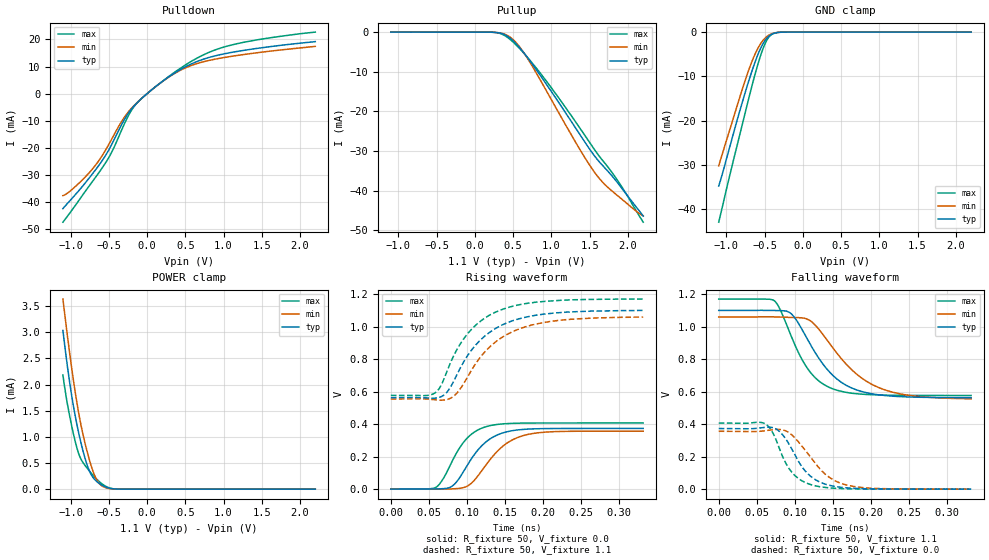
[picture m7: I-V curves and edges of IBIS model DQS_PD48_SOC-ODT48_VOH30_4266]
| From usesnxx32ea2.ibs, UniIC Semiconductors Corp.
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| DQS_PD48_SOC-ODT48_VOH30_4266
| (48 Ohm Pulldown, 48 Ohm System ODT Setting, VOH=VDDQ/3.0, 3200-4266Mbps)
[Model]   DQS_PD48_SOC-ODT48_VOH30_4266
Model_type   I/O
Vinl = 123.333mV
Vinh = 243.333mV
Vmeas = 183.333mV
Vref = 0.0mV
Cref = 0.0pF
Rref = 48.000Ohm
|   typ   min   max
|C_comp   0.849pF   0.799pF   0.899pF
C_comp_pullup   0.4245pF   0.3995pF   0.4495pF
C_comp_pulldown   0.4245pF   0.3995pF   0.4495pF
| Note: C_comp changes when the ODT circuit is enabled.
[Model Spec]
| Input threshold voltage corners
Vinl   0.1233V   0.1167V   0.1350V
Vinh   0.2433V   0.2367V   0.2550V
| Measurement voltage corners
Vmeas   0.1833V   0.1767V   0.1950V
| Timing spec test load voltage corners
Vref   0.0000V   0.0000V   0.0000V
| Dynamic Overshoot Parameters from LPDDR4 Specification
D_overshoot_ampl_h   0.30   NA   NA
D_overshoot_ampl_l   0.30   NA   NA
D_overshoot_area_h   0.1n   NA   NA
D_overshoot_area_l   0.1n   NA   NA
[Voltage Range]   1.1000V   1.0600V   1.1700V
[Pullup Reference]   1.1000V   1.0600V   1.1700V
| Junction Temperature (Ambient temp is 35C typ 95C min -40C max)
[Temperature Range]   50.0   110.0   -40.0
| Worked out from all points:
|   slope of the pulldown table from 0 to 0.165 V, typ, clamps not added: 43.9 ohm
|   slope of the pullup table from 0 to 0.165 V, typ, clamps not added: 15.7 kohm
|   GND clamp passes 1 mA (typ) near -0.45 V on its own axis
|   POWER clamp passes 1 mA (typ) near -0.88 V on its own axis
|   rising waveform, R_fixture 50, V_fixture 0.0: 20-80 % time 36.2ps typ, 40.6ps min, 31.9ps max; typ from 0.001 V to 0.373 V
|   falling waveform, R_fixture 50, V_fixture 1.1: 20-80 % time 49.2ps typ, 61ps min, 39.1ps max; typ from 1.1 V to 0.563 V
|   rising waveform, R_fixture 50, V_fixture 1.1: 20-80 % time 55.7ps typ, 58.6ps min, 51.8ps max; typ from 0.563 V to 1.1 V
|   falling waveform, R_fixture 50, V_fixture 0.0: 20-80 % time 32.4ps typ, 39.9ps min, 27.4ps max; typ from 0.373 V to 0.001 V
[Pulldown]
|   Voltage   I(typ)   I(min)   I(max)
-1.1V     -42.4mA    -37.62mA   -47.4mA
-911.9mV  -36.43mA   -33.59mA   -40.22mA
-680.9mV  -28.37mA   -26.64mA   -31.14mA
-482.9mV  -19.86mA   -17.85mA   -22.71mA
-314.6mV  -10.51mA   -9.476mA   -12.3mA
-176mV    -4.726mA   -4.587mA   -5.011mA
-47.3mV   -1.184mA   -1.177mA   -1.166mA
266.2mV   5.832mA    5.742mA    5.954mA
589.6mV   11.09mA    10.5mA     12.08mA
965.8mV   14.43mA    13.11mA    16.84mA
1.444V    16.71mA    15.1mA     19.86mA
2.2V      19.18mA    17.44mA    22.7mA
[GND Clamp]
|   Voltage   I(typ)   I(min)   I(max)
-1.1V     -34.74mA   -30.2mA    -42.91mA
-948.2mV  -25.43mA   -21.63mA   -31.79mA
-796.4mV  -16.11mA   -13.14mA   -21.19mA
-723.8mV  -11.93mA   -9.348mA   -16.1mA
-661.1mV  -8.566mA   -6.435mA   -11.85mA
-588.5mV  -5.112mA   -3.681mA   -7.299mA
-522.5mV  -2.666mA   -1.902mA   -3.81mA
-469.7mV  -1.356mA   -992.7uA   -1.786mA
-413.6mV  -564.8uA   -417.5uA   -621.5uA
-350.9mV  -166uA     -126.7uA   -147.9uA
-235.4mV  -8.3uA     -7.759uA   -4.464uA
2.2V      0A         0A         0A
[Pullup]
|   Voltage   I(typ)   I(min)   I(max)
-1.1V     5.229uA    8.059uA    2.358uA
233.2mV   -40.23uA   -40.58uA   -42.16uA
335.5mV   -284.9uA   -236.8uA   -392.1uA
437.8mV   -1.202mA   -984.9uA   -1.513mA
546.7mV   -3.115mA   -2.853mA   -3.399mA
675.4mV   -6.14mA    -6.273mA   -6.112mA
985.6mV   -14.62mA   -16.59mA   -13.71mA
1.388V    -26.34mA   -30.16mA   -24.7mA
1.596V    -32.06mA   -36.23mA   -30.58mA
1.698V    -34.29mA   -38.48mA   -33.08mA
1.873V    -38.23mA   -41.42mA   -37.69mA
2.2V      -46.44mA   -46.37mA   -47.99mA
[POWER Clamp]
|   Voltage   I(typ)   I(min)   I(max)
-1.1V     3.033mA    3.633mA    2.184mA
-1.041V   2.345mA    2.929mA    1.625mA
-961.4mV  1.581mA    2.073mA    1.051mA
-898.7mV  1.11mA     1.498mA    702.2uA
-845.9mV  780uA      1.103mA    527.5uA
-773.3mV  421uA      665.2uA    384.1uA
-710.6mV  232.4uA    359uA      273.1uA
-651.2mV  138.6uA    162.3uA    181.2uA
-591.8mV  77.92uA    64.83uA    105.5uA
-492.8mV  18.89uA    11.59uA    24.06uA
-374mV    1.385uA    999.3nA    1.123uA
2.2V      0A         0A         0A
[Ramp]
|   typ   min   max
| 20% - 80%
dV/dt_r   223.68m/36.23p   213.63m/40.56p   243.93m/31.88p
dV/dt_f   322.10m/49.17p   302.15m/60.99p   355.98m/39.04p
| 25% - 75%
|dV/dt_r   186.40m/28.84p   178.03m/32.35p   203.28m/25.32p
|dV/dt_f   268.41m/39.20p   251.79m/48.64p   296.65m/31.09p
R_load = 50
[Rising Waveform]
R_fixture = 50
V_fixture = 0.0
|   Time   V(typ)   V(min)   V(max)
0s        514.6uV    443.3uV    375.2uV
58ps      529.3uV    148.2uV    8.033mV
67ps      2.308mV    -205.7uV   50.16mV
79ps      13.47mV    1.162mV    155.5mV
91ps      73.54mV    5.154mV    257.6mV
103ps     164.9mV    25.41mV    325.6mV
127ps     297.2mV    160.2mV    386.4mV
151ps     350.9mV    277.1mV    402.6mV
181ps     369.4mV    337.2mV    406.4mV
332ps     373.3mV    356.5mV    406.9mV
[Falling Waveform]
R_fixture   = 50
V_fixture   = 1.1
V_fixture_min = 1.06
V_fixture_max = 1.17
|   Time   V(typ)   V(min)   V(max)
0s        1.1V       1.06V      1.17V
73ps      1.1V       1.06V      1.16V
81ps      1.099V     1.059V     1.104V
95ps      1.081V     1.057V     945.8mV
116ps     928.5mV    1.047V     748.2mV
131ps     810.4mV    988.5mV    668.6mV
150ps     700.9mV    870mV      617.7mV
181ps     611.6mV    709.7mV    587.5mV
215ps     578.2mV    617mV      579.2mV
332ps     563.2mV    556.4mV    576.7mV
[Rising Waveform]
R_fixture   = 50
V_fixture   = 1.1
V_fixture_min = 1.06
V_fixture_max = 1.17
|   Time   V(typ)   V(min)   V(max)
0s        562.8mV    553.9mV    576.6mV
57ps      559.1mV    550mV      588.5mV
66ps      568.1mV    547.2mV    637.4mV
79ps      631.5mV    560.2mV    783.2mV
91ps      741.5mV    614.4mV    890.5mV
109ps     871.9mV    753.3mV    996.5mV
126ps     950.3mV    855.7mV    1.059V
145ps     1.006V     929.5mV    1.103V
209ps     1.08V      1.031V     1.157V
332ps     1.099V     1.058V     1.169V
[Falling Waveform]
R_fixture = 50
V_fixture = 0.0
|   Time   V(typ)   V(min)   V(max)
0s        373.4mV    356.6mV    407mV
58ps      379.5mV    358.1mV    408.5mV
75ps      371.8mV    367.9mV    309.2mV
86ps      323.5mV    362.8mV    180.3mV
96ps      248.6mV    334.7mV    105.5mV
110ps     134.8mV    262mV      50.4mV
125ps     65.05mV    171.7mV    23.27mV
147ps     22.63mV    68.08mV    7.787mV
175ps     6.401mV    19.06mV    2.191mV
332ps     585.3uV    565.4uV    398.2uV
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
